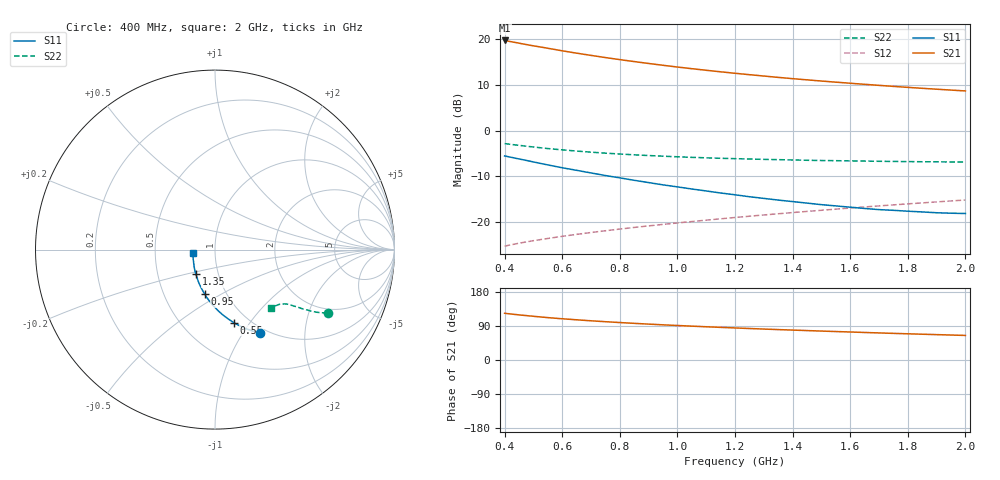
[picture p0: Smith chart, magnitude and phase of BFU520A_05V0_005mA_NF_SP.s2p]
! Filename:  P:\Prog\Test\Noise\ATS_data\Testdata_Net\06 Compressed Noise after Statistics\BFU520A_APG2013_30_A05_05p0V_005mA_NF_CM01_D.sf
! Date/Time: Wed 24/Apr/2013 20:06:18
! BFU520A_APG2013_30_A05_05p0V_1to20mA_NF_CM01_Bias4_R.sf
! Noise Parameter Data File
! BFU520A_APG2013_30_A05_05p0V_1to20mA_NF_CM01
! Date/time: Thu Apr 11 01:07:08 2013
! VAR V_out= 5.001000
! VAR I_out= 4.995000
! VAR V_in= 0.829300
! VAR I_in= 0.054605
! Device data file deembeded for feedlines and parallel
! Original file: \06 Compressed Noise after Statistics\BFU520A_APG2013_30_A05_05p0V_005mA_NF_CM01_R.sf
! Feed-files: PR017V01_150413_Feed1.s2p, PR017V01_150413_Feed2.s2p
! Parallel-file: PR017V01_150413_Par.s2p
# MHz S MA R 50
!  Freq-MHz  S11-mag  S11-arg  S21-mag  S21-arg  S12-mag  S12-arg  S22-mag  S22-arg
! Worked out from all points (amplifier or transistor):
!   37 points, 400 MHz to 2 GHz, reference 50 ohm
!   highest |S21| = 19.7 dB at 400 MHz (marker M1)
!   |S21| within 3 dB of that: start of sweep to 672.6 MHz
!   unconditionally stable (mu >= 1): 1.62 GHz to end of sweep
!   at 500 MHz: K = 0.63, MSG = 21.3 dB, |S12| = -24.1 dB
!   at 1.1 GHz: K = 0.93, MSG = 16.4 dB, |S12| = -19.6 dB
!   at 2 GHz: K = 1.01, MAG = 11.3 dB, |S12| = -15.2 dB
!   lowest NFmin = 0.66 dB at 420 MHz
!   S11 on the Smith chart (normalised r, x): 400 MHz: 0.93, -1.20; 550 MHz: 0.85, -0.84; 950 MHz: 0.79, -0.42; 1.35 GHz: 0.78, -0.22; 2 GHz: 0.78, -0.03
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400  0.5278 -61.5  9.673 123.3  0.05433 64.6  0.7195 -29.4
420  0.5117 -63.6  9.409 121.5  0.05607 64.2  0.7065 -30.0
440  0.4961 -65.6  9.162 119.9  0.0577 63.9  0.6944 -30.5
480  0.4678 -69.4  8.672 116.8  0.06081 63.4  0.671 -31.4
500  0.4536 -71.2  8.45 115.4  0.06239 63.2  0.6609 -31.8
550  0.4205 -75.5  7.947 111.8  0.06596 62.8  0.6352 -32.6
600  0.3917 -79.5  7.453 108.8  0.0696 62.7  0.6146 -33.2
650  0.3672 -83.0  7.024 106.1  0.07314 62.6  0.5964 -33.9
700  0.3436 -86.7  6.641 103.5  0.07663 62.7  0.5802 -34.3
750  0.3221 -90.0  6.284 101.1  0.0801 62.8  0.5658 -34.7
800  0.3035 -93.5  5.97 98.8  0.0836 63.0  0.5537 -35.1
850  0.2856 -96.7  5.681 96.7  0.08707 63.1  0.5425 -35.5
900  0.2697 -100.0  5.419 94.7  0.09057 63.3  0.5328 -35.9
950  0.2545 -103.0  5.174 92.8  0.09403 63.5  0.5239 -36.1
1050  0.2293 -109.1  4.75 89.3  0.101 63.9  0.5088 -36.8
1100  0.2183 -112.2  4.564 87.7  0.1046 64.1  0.503 -37.1
1200  0.1983 -118.3  4.232 84.6  0.1119 64.4  0.4923 -37.9
1350  0.1735 -127.8  3.816 80.2  0.1229 64.8  0.4803 -39.1
1500  0.1546 -137.8  3.481 76.4  0.1342 65.0  0.4701 -40.5
1650  0.1405 -147.8  3.205 72.7  0.1459 65.1  0.4635 -42.1
1750  0.134 -154.9  3.042 70.3  0.1537 65.1  0.4591 -43.1
2000  0.1237 -172.1  2.712 64.8  0.1738 64.8  0.4519 -46.2
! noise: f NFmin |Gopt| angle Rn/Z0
400  0.6869  0.1988  14.59  0.1319
460  0.6774  0.1799  19.48  0.1226
600  0.758  0.2135  18.24  0.1503
800  0.7422  0.1594  44.88  0.1107
1000  0.7631  0.1609  55.96  0.1072
1200  0.7989  0.1489  70.95  0.1052
1400  0.8581  0.1297  86.78  0.0953
1600  0.8387  0.1087  102.5  0.095
1800  0.8192  0.1152  128.3  0.0864
2000  0.8528  0.1088  143.5  0.0858
